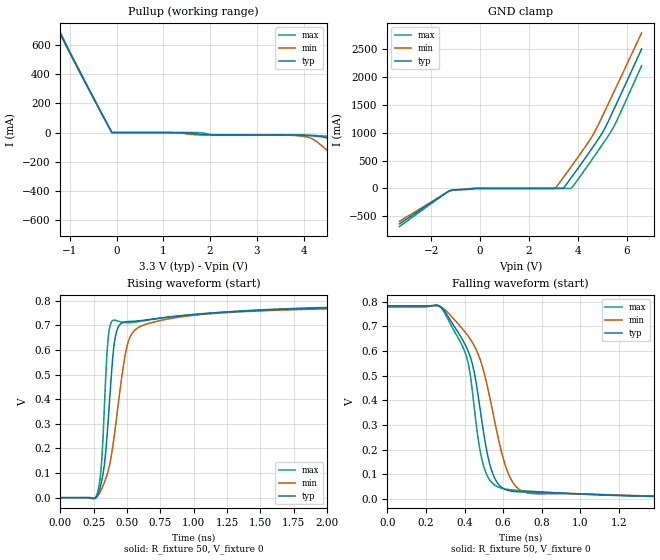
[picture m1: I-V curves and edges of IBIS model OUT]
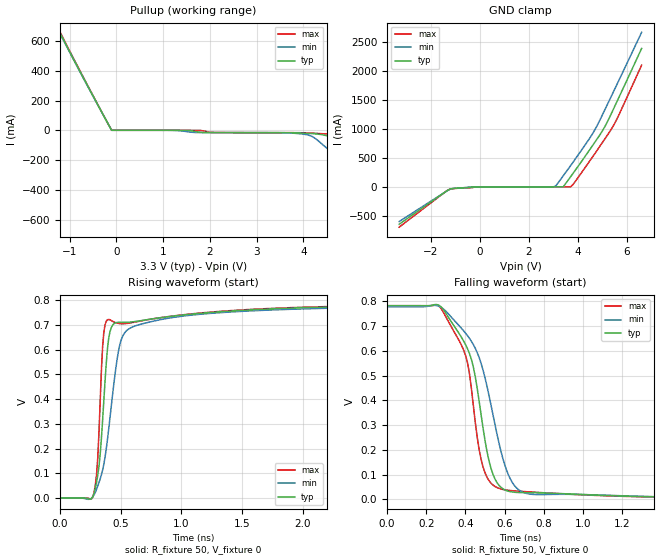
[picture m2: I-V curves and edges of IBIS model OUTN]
|   IBIS File of SG2520HHN C
|   HCSL Zdiff=100, Vcc=3.3V, fo>212.5MHz
[IBIS Ver]   3.2
[File Name]   sg2520hhn_hf_33v.ibs
[File Rev]   1.0
[Date]   Aug. 4, 2020
[Source]
[Notes]
Created by Minoru Kozaki
[Disclaimer]
Seiko Epson Corporation makes no warranty with respect to the
information contained herein.
[Copyright]
Copyright(C) 2020, Seiko Epson Corporation. All rights reserved.
|   Component
[Component]   SG2520HHN
[Manufacturer]  Seiko Epson Corporation
[Package]
R_pkg   17.7m   NA   NA
L_pkg   235p   NA   NA
C_pkg   208f   NA   NA
[Pin]   signal_name   model_name   R_pin   L_pin   C_pin
1   OE/ST   NC
2   NC   NC
3   GND   GND
4   OUT   OUT   17.7m   235p   208f
5   OUTN   OUTN   10.4m   129p   221f
6   VCC   POWER
[Diff Pin] inv_pin  vdiff  tdelay_typ
4   5   0   0
| Models and submodels in the file (2): OUT (Open_source), OUTN (Open_source)
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|   Model OUT
[Model]   OUT
Model_type   Open_source
Polarity   Non-Inverting
Vref = 0
Vmeas = 0.4
Rref = 50
Cref = 0
C_comp   12.0p   12.0p   12.0p
[Temperature Range]   25   105   -40
[Voltage Range]   3.3   2.97   3.63
[Pullup Reference]   3.3   2.97   3.63
[GND Clamp Reference]   0   0   0
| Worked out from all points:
|   GND clamp passes 1 mA (typ) near -0.23 V on its own axis
|   falling waveform, R_fixture 50, V_fixture 0: 20-80 % time 123ps typ, 154ps min, 106ps max; typ from 0.783 V to 0 V
|   rising waveform, R_fixture 50, V_fixture 0: 20-80 % time 70ps typ, 126ps min, 44.2ps max; typ from 0 V to 0.782 V
[Pullup]
-3.3V     2.51A      2.488A     2.534A
-1.3V     738.6mA    733.7mA    747.2mA
-1.2V     675.3mA    670.8mA    683mA
-100mV    32.53uA    19.73uA    91.95uA
1.7V      -8.605mA   -15.11mA   -82.95uA
3.9V      -17.97mA   -22.6mA    -16.25mA
4.2V      -22.5mA    -43.64mA   -19.36mA
4.5V      -36.89mA   -119.5mA   -25.2mA
4.6V      -54.67mA   -146.2mA   -27.99mA
4.8V      -112mA     -199.5mA   -36.77mA
5V        -170.4mA   -253mA     -73.63mA
6.6V      -638.6mA   -681.9mA   -581.5mA
[GND Clamp]
-3.3V     -637.9mA   -592.2mA   -686.6mA
-1.4V     -81.81mA   -84.3mA    -81.62mA
-1.2V     -36.02mA   -38.45mA   -37.51mA
-100mV    -30.13uA   -15.99uA   -185.8uA
3.1V      -1.477uA   17.81mA    -3.233uA
3.4V      32.53uA    197.2mA    -2.45uA
3.7V      179.9mA    378.5mA    30.97uA
3.8V      240.6mA    440.1mA    41.86mA
4.6V      738.6mA    954.1mA    535.8mA
5V        1.004A     1.302A     792.3mA
5.5V      1.455A     1.767A     1.142A
6.6V      2.51A      2.798A     2.208A
[Falling Waveform]
R_fixture = 50
V_fixture = 0
V_fixture_min = 0
V_fixture_max = 0
0s        783.4mV    778.7mV    783.3mV
270ps     783.4mV    780.9mV    781.9mV
420ps     597.5mV    659.2mV    547.6mV
450ps     514.1mV    621.8mV    372.1mV
470ps     421mV      588.3mV    245.5mV
500ps     261.7mV    515.3mV    129.5mV
550ps     93.9mV     337.6mV    59.26mV
630ps     32.83mV    96.12mV    37.2mV
770ps     26.88mV    20.09mV    28.9mV
4ns       242uV      318uV      228uV
[Rising Waveform]
R_fixture = 50
V_fixture = 0
V_fixture_min = 0
V_fixture_max = 0
0s        98uV       123uV      104uV
280ps     10.33mV    7.159mV    23.14mV
310ps     68.57mV    36.23mV    150.1mV
340ps     186mV      76.91mV    493.6mV
360ps     325.8mV    112mV      658.7mV
400ps     609.6mV    235.2mV    720.8mV
440ps     698.2mV    406.2mV    715.6mV
510ps     715.2mV    634.5mV    710.5mV
670ps     723.6mV    708.6mV    722.2mV
4ns       782.4mV    777.4mV    782.5mV
[Ramp]
R_load = 50
dV/dt_r   0.47246/69.96p   0.46893/127.34p   0.47298/43.95p
dV/dt_f   0.47246/124.33p   0.46893/155.49p   0.47298/108.12p
|   Model OUTN
[Model]   OUTN
Model_type   Open_source
Polarity   Inverting
Vref = 0
Vmeas = 0.4
Rref = 50
Cref = 0
C_comp   12.0p   12.0p   12.0p
[Temperature Range]   25   105   -40
[Voltage Range]   3.3   2.97   3.63
[Pullup Reference]   3.3   2.97   3.63
[GND Clamp Reference]   0   0   0
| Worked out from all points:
|   GND clamp passes 1 mA (typ) near -0.23 V on its own axis
|   falling waveform, R_fixture 50, V_fixture 0: 20-80 % time 120ps typ, 152ps min, 103ps max; typ from 0.783 V to 0 V
|   rising waveform, R_fixture 50, V_fixture 0: 20-80 % time 69.7ps typ, 127ps min, 43.4ps max; typ from 0 V to 0.782 V
[Pullup]
-3.3V     2.385A     2.367A     2.405A
-1.3V     712.9mA    708.1mA    721mA
-1.2V     651.7mA    647.5mA    659mA
-100mV    32.53uA    19.73uA    91.96uA
3.9V      -17.97mA   -22.59mA   -16.25mA
4.2V      -22.49mA   -43.67mA   -19.36mA
4.5V      -36.9mA    -120.3mA   -25.2mA
4.6V      -54.84mA   -147.3mA   -27.99mA
4.8V      -112.8mA   -201.2mA   -36.79mA
4.9V      -142.4mA   -228.2mA   -48.29mA
5V        -171.9mA   -255.2mA   -74.16mA
6.6V      -645.5mA   -688.6mA   -588.4mA
[GND Clamp]
-3.3V     -644.9mA   -598mA     -694.8mA
-1.4V     -82.36mA   -84.78mA   -82.3mA
-1.2V     -36.03mA   -38.45mA   -37.55mA
-100mV    -30.13uA   -15.99uA   -185.7uA
3.1V      -1.477uA   17.19mA    -3.233uA
3.4V      32.53uA    190.3mA    -2.45uA
3.7V      173.6mA    365.3mA    30.97uA
4.3V      529.7mA    726.4mA    336.1mA
4.7V      774.2mA    989.6mA    578.5mA
5V        965.1mA    1.241A     764.5mA
5.5V      1.385A     1.683A     1.093A
6.6V      2.385A     2.662A     2.096A
[Falling Waveform]
R_fixture = 50
V_fixture = 0
V_fixture_min = 0
V_fixture_max = 0
0s        782.9mV    778.2mV    782.7mV
270ps     782.1mV    778.7mV    777.1mV
380ps     654.4mV    690.9mV    622.6mV
420ps     590.3mV    651.1mV    510.2mV
460ps     448mV      593.4mV    250mV
490ps     286.3mV    521.3mV    130mV
540ps     101.7mV    342.9mV    58.18mV
620ps     32.69mV    97.16mV    36.52mV
760ps     26.65mV    19.55mV    28.68mV
4ns       238uV      309uV      224uV
[Rising Waveform]
R_fixture = 50
V_fixture = 0
V_fixture_min = 0
V_fixture_max = 0
0s        93uV       127uV      102uV
280ps     19.46mV    13.09mV    23.62mV
310ps     91.3mV     48.84mV    160.9mV
350ps     313mV      112.6mV    609.8mV
390ps     602.2mV    235.9mV    720.2mV
430ps     696.6mV    407.3mV    714.7mV
500ps     710.3mV    633.6mV    704.3mV
640ps     714.6mV    698.7mV    713mV
1.6ns     760.7mV    756.7mV    762.7mV
4ns       781.7mV    776.7mV    781.9mV
[Ramp]
R_load = 50
dV/dt_r   0.47242/69.56p   0.46890/127.93p   0.47293/43.53p
dV/dt_f   0.47242/122.06p   0.46890/153.39p   0.47293/105.77p
